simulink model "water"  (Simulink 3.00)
settings: Solver=ode1  SolverMode=SingleTasking  StartTime=0.0  StopTime=inf  FixedStep=.5  RelTol=1e-3  AbsTol=1e-6
PreLoadFcn:
  | watergui
StartFcn:
  | watergui start
StopFcn:
  | watergui stop
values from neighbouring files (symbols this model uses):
  area = 100    [watergui.m]
  hilim = evalin('base','hilim')    [watergui.m]
  inflow = 10    [watergui.m]
  lolim = evalin('base','lolim')    [watergui.m]
  outflow = 40    [watergui.m]

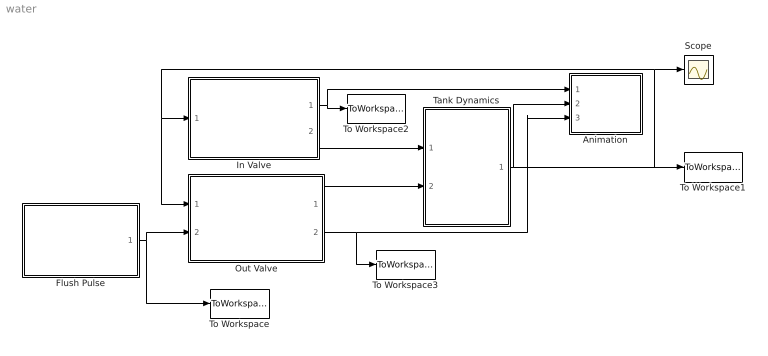
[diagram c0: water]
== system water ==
  Animation : Subsystem
  Flush Pulse : Subsystem
  In Valve : Subsystem  mask{hilim=hilim, inflow=inflow}
      mask prompts: hilim "Shut Off Height"; inflow "Flow Rate"
  Out Valve : Subsystem
  Scope : Scope
  Tank Dynamics : Subsystem
  To Workspace : ToWorkspace  VariableName=flushpulse  SampleTime=-1  SaveFormat=Matrix
  To Workspace1 : ToWorkspace  VariableName=tankheight  SampleTime=-1  SaveFormat=Matrix
  To Workspace2 : ToWorkspace  VariableName=invalve  SampleTime=-1  SaveFormat=Matrix
  To Workspace3 : ToWorkspace  VariableName=Outvalve  SampleTime=-1  SaveFormat=Matrix
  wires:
  Out Valve/2(Valve Position) -> Animation/3(Outvalve), To Workspace3/1
  In Valve/1(Valve Position) -> Animation/1(In Valve), To Workspace2/1
  Tank Dynamics/1(Tank Height) -> Scope/1, Out Valve/1(Tank Height), In Valve/1(Tank Height), Animation/2(Water Height), To Workspace1/1
  In Valve/2(ValveFlow) -> Tank Dynamics/1(Tank Inflow)
  Flush Pulse/1(Flush Signal) -> Out Valve/2(Flush Signal), To Workspace/1
  Out Valve/1(Flow Rate - Out) -> Tank Dynamics/2(Tank Outflow)

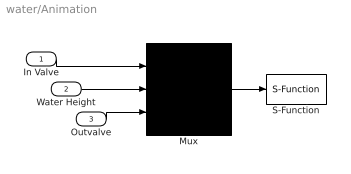
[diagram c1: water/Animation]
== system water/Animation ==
  In Valve : Inport  Port=1  PortWidth=-1  SampleTime=-1  DataType=auto
  Water Height : Inport  Port=2  PortWidth=-1  SampleTime=-1  DataType=auto
  Outvalve : Inport  Port=3  PortWidth=-1  SampleTime=-1  DataType=auto
  Mux : Mux  Inputs=3
  S-Function : S-Function  FunctionName=watersfun  Parameters=inflow,outflow,lolim,hilim,area  PortCounts=[]  SFunctionModules=''
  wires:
  Outvalve/1 -> Mux/3
  Water Height/1 -> Mux/2
  Mux/1 -> S-Function/1
  In Valve/1 -> Mux/1

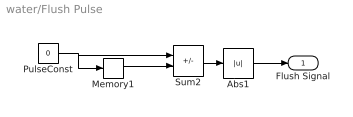
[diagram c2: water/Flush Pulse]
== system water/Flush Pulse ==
  Abs1 : Abs
  Memory1 : Memory  X0=0  InheritSampleTime=off
  PulseConst : Constant  Value=0
  Sum2 : Sum  Inputs=+-  SaturateOnIntegerOverflow=on
  Flush Signal : Outport  Port=1  InitialOutput=0
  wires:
  PulseConst/1 -> Sum2/1, Memory1/1
  Sum2/1 -> Abs1/1
  Memory1/1 -> Sum2/2
  Abs1/1 -> Flush Signal/1

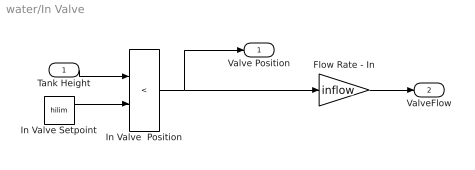
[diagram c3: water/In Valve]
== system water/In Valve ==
  Tank Height : Inport  Port=1  PortWidth=-1  SampleTime=-1  DataType=auto
  Flow Rate - In : Gain  Gain=inflow  SaturateOnIntegerOverflow=on
  In Valve  Position : RelationalOperator  Operator=<
  In Valve Setpoint : Constant  Value=hilim
  Valve Position : Outport  Port=1  InitialOutput=0
  ValveFlow : Outport  Port=2  InitialOutput=0
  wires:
  Flow Rate - In/1 -> ValveFlow/1
  In Valve  Position/1 -> Flow Rate - In/1, Valve Position/1
  Tank Height/1 -> In Valve  Position/1
  In Valve Setpoint/1 -> In Valve  Position/2

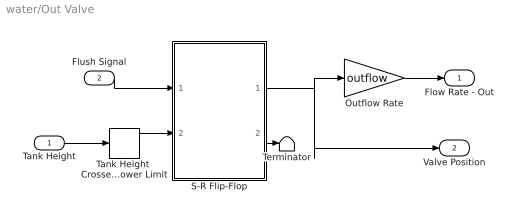
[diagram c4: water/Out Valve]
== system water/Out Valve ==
  Tank Height : Inport  Port=1  PortWidth=-1  SampleTime=-1  DataType=auto
  Flush Signal : Inport  Port=2  PortWidth=-1  SampleTime=-1  DataType=auto
  Outflow Rate : Gain  Gain=outflow  SaturateOnIntegerOverflow=on
  S-R Flip-Flop : Subsystem
  Tank Height  Crosses Lower Limit : HitCross  HitCrossingOffset=lolim  HitCrossingDirection=falling  ShowOutputPort=on
  Terminator : Terminator
  Flow Rate - Out : Outport  Port=1  InitialOutput=0
  Valve Position : Outport  Port=2  InitialOutput=0
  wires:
  Tank Height/1 -> Tank Height  Crosses Lower Limit/1
  Tank Height  Crosses Lower Limit/1 -> S-R Flip-Flop/2(R)
  S-R Flip-Flop/1(Q) -> Outflow Rate/1, Valve Position/1
  Flush Signal/1 -> S-R Flip-Flop/1(S)
  S-R Flip-Flop/2(!Q) -> Terminator/1
  Outflow Rate/1 -> Flow Rate - Out/1

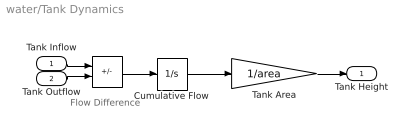
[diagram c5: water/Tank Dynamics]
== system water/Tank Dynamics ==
  note: Flow Difference
  Tank Inflow : Inport  Port=1  PortWidth=-1  SampleTime=-1  DataType=auto
  Tank Outflow : Inport  Port=2  PortWidth=-1  SampleTime=-1  DataType=auto
  " " : Sum  Inputs=+-  SaturateOnIntegerOverflow=on
  Cumulative Flow : Integrator  ExternalReset=none  InitialConditionSource=internal  InitialCondition=(hilim+lolim)/2*area  LimitOutput=off  UpperSaturationLimit=inf  LowerSaturationLimit=-inf  ShowSaturationPort=off  ShowStatePort=off  AbsoluteTolerance=auto
  Tank Area : Gain  Gain=1/area  SaturateOnIntegerOverflow=on
  Tank Height : Outport  Port=1  InitialOutput=0
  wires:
  Tank Outflow/1 -> " "/2
  Tank Inflow/1 -> " "/1
  " "/1 -> Cumulative Flow/1
  Cumulative Flow/1 -> Tank Area/1
  Tank Area/1 -> Tank Height/1

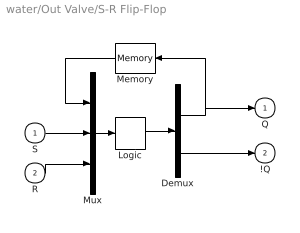
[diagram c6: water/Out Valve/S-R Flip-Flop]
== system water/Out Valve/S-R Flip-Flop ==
  S : Inport  Port=1  PortWidth=-1  SampleTime=-1  DataType=auto
  R : Inport  Port=2  PortWidth=-1  SampleTime=-1  DataType=auto
  Demux : Demux  Outputs=2
  Logic : CombinatorialLogic  TruthTable=[0 1;0 1;1 0;0 1;1 0;0 1;1 0;1 0]
  Memory : Memory  Orientation=left  X0=0  InheritSampleTime=on
  Mux : Mux  Inputs=3
  Q : Outport  Port=1  InitialOutput=0
  !Q : Outport  Port=2  InitialOutput=1
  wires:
  R/1 -> Mux/3
  S/1 -> Mux/2
  Memory/1 -> Mux/1
  Demux/1 -> Memory/1, Q/1
  Demux/2 -> !Q/1
  Logic/1 -> Demux/1
  Mux/1 -> Logic/1
